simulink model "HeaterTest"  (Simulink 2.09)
settings: Solver=ode45  StartTime=0.0  StopTime=20  MaxStep=10  RelTol=1e-3  AbsTol=1e-3
undefined symbols (not defined in the file or in its folder): sfunyst
libraries: fuzzy x1

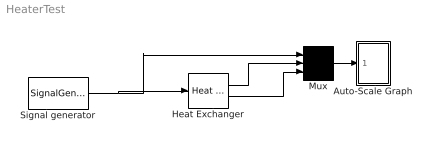
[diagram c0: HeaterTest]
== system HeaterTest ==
  Auto-Scale Graph : Subsystem  mask(Storage scope.){}
      mask help: Storage scope using MATLAB graph window. Enter plotting ranges and line type.
      mask init:
      | npts = @4; color = @5; ax = [0, @1, @2, @3]; dt=@6;
  Heat Exchanger : fuzzy/Heat Exchanger
  Mux : Mux  Inputs=3
  Signal generator : SignalGenerator  WaveForm=square  Amplitude=1.000000  Frequency=0.5  Units=rad/sec
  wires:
  Heat Exchanger/2 -> Mux/3
  Heat Exchanger/1 -> Mux/2
  Signal generator/1 -> Heat Exchanger/1, Mux/1
  Mux/1 -> Auto-Scale Graph/1(x)

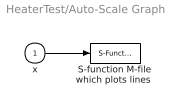
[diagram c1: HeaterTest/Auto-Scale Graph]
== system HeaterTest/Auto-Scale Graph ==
  x : Inport  Port=1  PortWidth=-1  SampleTime=-1
  "S-function M-file which plots lines " : S-Function  LoadFcn=sfunyst([],[],[],'LoadBlock')  FunctionName=sfunyst  Parameters=ax, color, npts, dt
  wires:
  x/1 -> "S-function M-file which plots lines "/1
